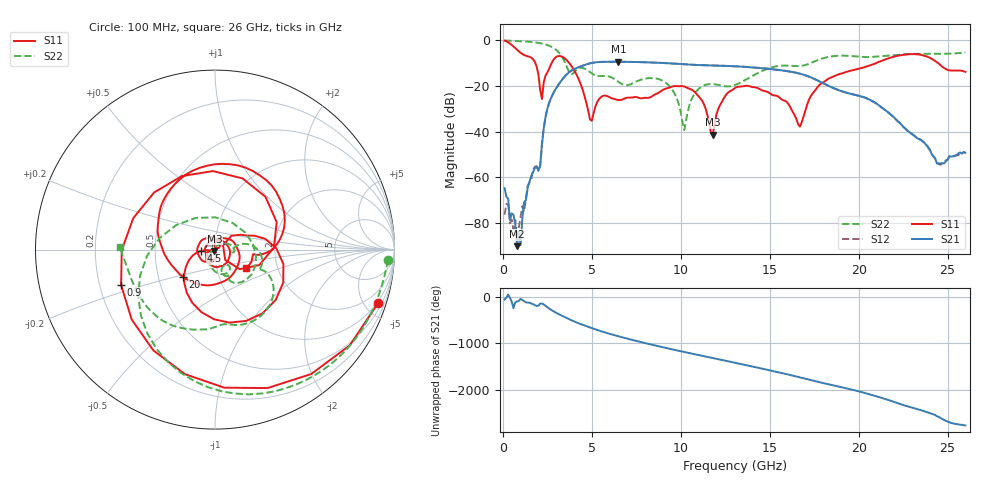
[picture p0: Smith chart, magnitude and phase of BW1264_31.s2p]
!Keysight Technologies,N5245B,MY57181159,A.13.60.06
!Date: Friday, December 18, 2020 23:53:34
!Correction: S11(Full 2 Port(1,2))
!S21(Full 2 Port(1,2))
!S12(Full 2 Port(1,2))
!S22(Full 2 Port(1,2))
!S2P File: Measurements: S11, S21, S12, S22:
# Hz S  dB  R 50
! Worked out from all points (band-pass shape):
!   260 points, 100 MHz to 26 GHz, reference 50 ohm
!   highest |S21| = -9.57 dB at 6.5 GHz (marker M1); lowest = -89.9 dB at 800 MHz (marker M2)
!   |S21| within 3 dB of the highest: 4.066 GHz to 14.84 GHz (10.78 GHz wide, 114 % of centre)
!   lowest |S11| = -41.3 dB at 11.8 GHz (marker M3), VSWR 1.02, Z = 49.7 - j0.803 ohm
!   |S11| at or under -10 dB: 1.817 GHz to 2.756 GHz (939.3 MHz wide, 41.1 % of centre); 3.718 GHz to 21.02 GHz (17.31 GHz wide, 140 % of centre); 24.43 GHz to end of sweep
!   |S22| runs from -39.4 to -0.3 dB; largest |S21 - S12| = 0.00057
!   S11 on the Smith chart (normalised r, x): 100 MHz: 0.88, -6.12; 900 MHz: 0.29, -0.17; 4.5 GHz: 0.86, -0.01; 20 GHz: 0.67, -0.21; 26 GHz: 1.37, -0.30
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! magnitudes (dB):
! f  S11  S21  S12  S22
! 100 MHz  -0.4  -64.6  -76.3  -0.3
! 400 MHz  -1.7  -78.6  -79.9  -0.4
! 800 MHz  -4.3  -89.9  -86.3  -0.6
! 900 MHz  -5.1  -83.9  -81.6  -0.6
! 1.8 GHz  -9.7  -56.0  -55.3  -1.1
! 2.2 GHz  -25.8  -45.6  -45.6  -1.6
! 2.7 GHz  -10.9  -25.6  -25.6  -2.9
! 3.5 GHz  -8.2  -15.8  -15.8  -10.0
! 4.5 GHz  -22.1  -11.3  -11.3  -12.3
! 5 GHz  -35.3  -10.1  -10.1  -14.7
! 6.5 GHz  -26.3  -9.6  -9.6  -18.4
! 8.8 GHz  -22.9  -10.0  -10.0  -17.3
! 10.2 GHz  -20.4  -10.7  -10.7  -39.4
! 10.7 GHz  -22.2  -10.9  -10.9  -24.5
! 11.8 GHz  -41.3  -11.2  -11.2  -19.3
! 13.1 GHz  -20.8  -11.6  -11.6  -19.5
! 16.7 GHz  -37.8  -14.8  -14.8  -11.5
! 17.4 GHz  -23.5  -16.7  -16.7  -9.8
! 20 GHz  -12.6  -24.4  -24.4  -7.4
! 21.7 GHz  -8.0  -31.9  -31.9  -6.9
! 24.4 GHz  -9.8  -53.9  -53.7  -6.1
! 26 GHz  -14.0  -49.2  -49.3  -5.5
